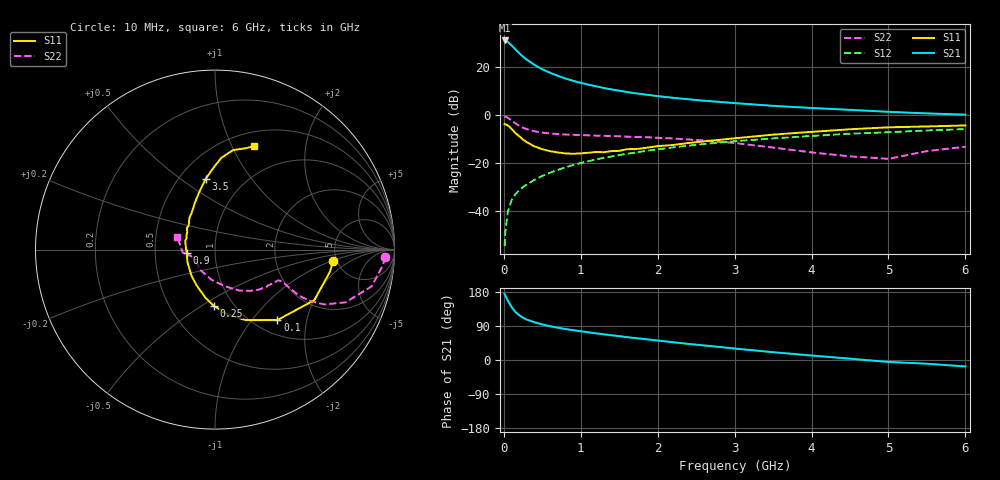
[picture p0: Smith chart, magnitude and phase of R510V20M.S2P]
! SIEMENS Small Signal Semiconductors
! BFR183
! Si NPN RF Bipolar Junction Transistor in SOT23
! VCE = 10 V  IC = 20 mA
! Common Emitter S-Parameters:  May  1996
# GHz  S  MA  R  50
!  f  S11  S21  S12  S22
! GHz  MAG  ANG  MAG  ANG  MAG  ANG  MAG  ANG
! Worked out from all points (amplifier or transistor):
!   36 points, 10 MHz to 6 GHz, reference 50 ohm
!   highest |S21| = 31.1 dB at 10 MHz (marker M1)
!   |S21| within 3 dB of that: start of sweep to 129.6 MHz
!   unconditionally stable (mu >= 1): 642.4 MHz to 2.608 GHz
!   at 250 MHz: K = 0.77, MSG = 27.1 dB, |S12| = -29.8 dB
!   at 1.4 GHz: K = 1.04, MAG = 12.7 dB, |S12| = -17.1 dB
!   at 6 GHz: K = 0.90, MSG = 3.0 dB, |S12| = -5.7 dB
!   S11 on the Smith chart (normalised r, x): 10 MHz: 4.68, -1.04; 100 MHz: 1.25, -1.35; 250 MHz: 0.81, -0.56; 900 MHz: 0.73, -0.03; 3.5 GHz: 0.67, +0.62; 6 GHz: 0.66, +1.22
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0.01  0.6624 -5.4  36.05 174.3  0.0019 83.3  0.9484 -2.5
0.02  0.6518 -11.0  35.77 169.7  0.0038 75.4  0.939 -5.4
0.05  0.6212 -26.9  33.82 157.3  0.0096 74.9  0.8963 -13.2
0.1  0.5244 -48.5  28.57 140.0  0.0172 70.8  0.7844 -22.0
0.15  0.4287 -66.5  23.61 126.6  0.0229 67.5  0.6806 -26.7
0.2  0.3666 -79.2  19.65 118.1  0.0279 67.2  0.6059 -28.3
0.25  0.3125 -91.4  16.56 111.5  0.0324 67.6  0.5522 -28.7
0.3  0.2743 -101.0  14.3 106.4  0.0367 68.1  0.5142 -28.3
0.4  0.2256 -116.5  11.17 99.6  0.0456 69.2  0.4646 -27.2
0.5  0.1971 -131.3  9.057 93.8  0.0548 69.8  0.4373 -26.3
0.6  0.1796 -142.1  7.669 89.2  0.0642 69.8  0.4202 -25.7
0.7  0.169 -154.8  6.646 85.3  0.0734 70.1  0.4086 -25.6
0.9  0.1584 -173.6  5.214 78.7  0.0926 69.5  0.3924 -25.9
1.1  0.1665 170.3  4.341 73.1  0.1114 68.4  0.3832 -27.7
1.3  0.1709 158.0  3.7 67.8  0.1303 66.8  0.3738 -29.4
1.6  0.1975 142.4  3.055 60.3  0.1586 64.0  0.36 -33.2
2.2  0.2413 123.0  2.311 46.9  0.2152 58.0  0.3301 -42.5
3.5  0.3963 97.6  1.575 20.6  0.3311 42.0  0.2135 -74.1
4.5  0.513 86.0  1.3 3.5  0.4145 29.8  0.1401 -126.0
5  0.5629 79.8  1.182 -5.2  0.4452 22.6  0.1244 -159.8
5.5  0.5869 73.8  1.096 -9.8  0.4837 18.6  0.1804 -174.6
6  0.6156 69.2  1.031 -17.0  0.5174 11.3  0.2221 160.9
